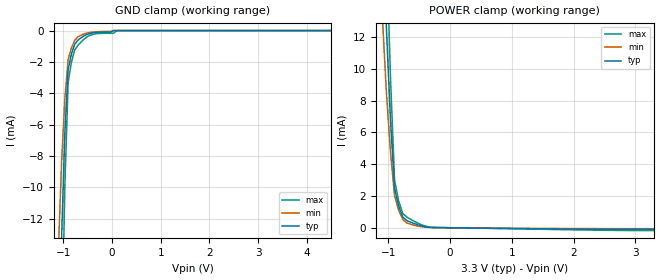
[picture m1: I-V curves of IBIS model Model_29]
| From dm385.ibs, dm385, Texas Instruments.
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| Model based on original model for IQ1833DVTCKPBFBP18LL_SSDHH
|   Sub model IQ_SSDHH_PU_ON_5P_3P3
[model]   Model_29
|[Description]  [3.3V-INPUT-PU-X, IND, 5%]
|   Weak internal pull-up,Industrial temperature range (-40C to
|   125C, 25C nominal),5% power supply tolerance
|[Input Load]   PU
|[Output Drive]
|Voltage   3.3V
|Mode   INPUT
Model_type   Input
Polarity   Non-Inverting
Vinl =  0.8V
Vinh =  2V
C_comp   1.115166p   0.9969108p   1.462567p
[Model Spec]
Vinl   0.8V   0.8V   0.8V
Vinh   2V   2V   2V
[Temperature Range]   25   125   -40
[Voltage Range]   3.3   3.135   3.465
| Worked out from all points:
|   GND clamp passes 1 mA (typ) near -0.78 V on its own axis
|   POWER clamp passes 1 mA (typ) near -0.80 V on its own axis
[POWER_clamp]
-3.3V     372.1mA    388.5mA    506.4mA
-1.1V     20.1mA     13.48mA    29.14mA
-1.033V   12.7mA     8.617mA    18.25mA
-966.7mV  6.831mA    4.797mA    9.545mA
-900mV    2.493mA    2.019mA    3.013mA
-833.3mV  1.353mA    1.101mA    1.678mA
-766.7mV  674.6uA    528.5uA    898.2uA
-700mV    455.9uA    301.6uA    672.6uA
-500mV    162.9uA    94.87uA    253.4uA
-300mV    23.19uA    14.14uA    37.02uA
3.3V      -100.3uA   -54.44uA   -173uA
[GND_clamp]
-3.3V     -586.5mA   -522.8mA   -870.8mA
-1.1V     -22.37mA   -13.97mA   -35.2mA
-1.033V   -13.09mA   -8.34mA    -20.44mA
-966.7mV  -6.465mA   -4.3mA     -9.807mA
-900mV    -2.481mA   -1.85mA    -3.307mA
-833.3mV  -1.501mA   -1.117mA   -2.022mA
-766.7mV  -878uA     -631.5uA   -1.238mA
-633.3mV  -455.6uA   -289.1uA   -727.4uA
-433.3mV  -176.8uA   -114.8uA   -285.2uA
33.33mV   0A         0A         -174uA
100mV     0A         0A         0A
6.6V      0A         0A         0A
